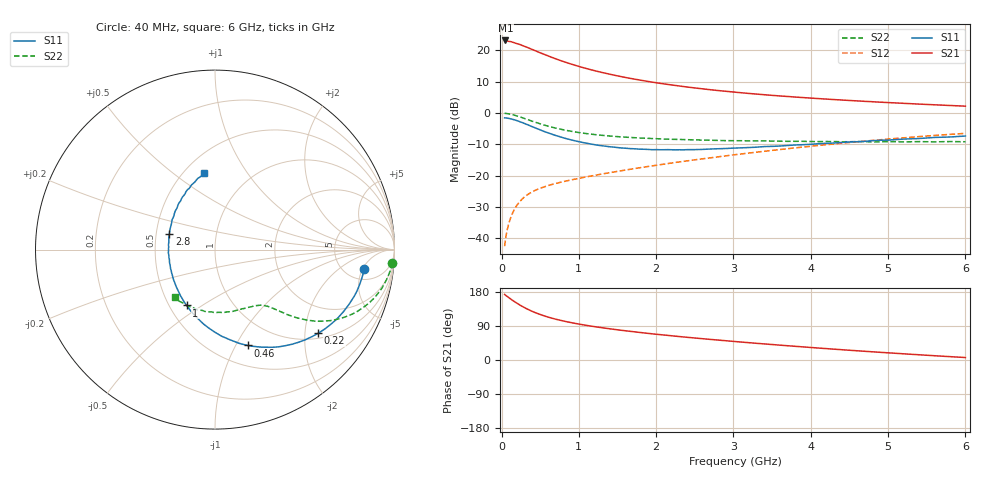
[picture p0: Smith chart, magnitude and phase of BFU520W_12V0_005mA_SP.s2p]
! Filename:  P:\Prog\Test\Noise\ATS_data\Testdata_Net\Run2\BFU520W_APM2013_06_A05_12p0V_005mA_SP_CM01_D.s2p
! Date/Time: Tue 26/Mar/2013 18:01:43
! BFU520W_APM2013_06_A05_12p0V_1to20mA_SP_CM01_Bias4_R.s2p
! MDIF S-parameter v. bias file
! BFU520W_APM2013_06_A05_12p0V_1to20mA_SP_CM01
! Date/time Thu Mar 21 16:35:01 2013
! VAR V_out= 12.0010
! VAR I_out= 5.0050
! VAR V_in= 0.8122
! VAR I_in= 0.0494
! Device data file deembeded for feedlines and parallel
! Original file: \Run2\BFU520W_APM2013_06_A05_12p0V_005mA_SP_CM01_R.s2p
! Feed-files: PR019V01_070313_Feed1.s2p, PR019V01_070313_Feed2.s2p
! Parallel-file: PR019V01_070313_Par.s2p
# MHz S MA R 50
!  Freq-MHz  S11-mag  S11-arg  S21-mag  S21-arg  S12-mag  S12-arg  S22-mag  S22-arg
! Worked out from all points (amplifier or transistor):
!   98 points, 40 MHz to 6 GHz, reference 50 ohm
!   highest |S21| = 23.2 dB at 50 MHz (marker M1)
!   |S21| within 3 dB of that: start of sweep to 409.2 MHz
!   unconditionally stable (mu >= 1): 1.889 GHz to 3.053 GHz
!   at 300 MHz: K = 0.32, MSG = 24.0 dB, |S12| = -26.8 dB
!   at 1.6 GHz: K = 0.97, MSG = 14.8 dB, |S12| = -18.2 dB
!   at 6 GHz: K = 0.86, MSG = 4.3 dB, |S12| = -6.5 dB
!   S11 on the Smith chart (normalised r, x): 40 MHz: 7.33, -5.42; 220 MHz: 1.13, -2.34; 460 MHz: 0.71, -1.12; 1 GHz: 0.61, -0.43; 2.8 GHz: 0.59, +0.11; 6 GHz: 0.63, +0.65
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40  0.8386 -7.5  14.41 173.1  0.007489 83.9  0.9894 -4.3
50  0.836 -9.3  14.42 171.4  0.009267 83.6  0.9873 -5.5
60  0.8331 -11.2  14.2 169.7  0.01116 82.6  0.984 -6.7
120  0.8065 -22.2  13.81 160.7  0.02159 77.6  0.9552 -12.9
160  0.7831 -29.1  13.32 155.2  0.02801 74.2  0.929 -16.7
220  0.7405 -39.0  12.64 147.2  0.03645 70.0  0.8814 -21.8
260  0.7105 -45.1  12.11 142.4  0.04146 67.4  0.8494 -24.8
320  0.663 -53.9  11.35 135.8  0.04807 64.3  0.8 -28.6
380  0.6183 -61.6  10.55 130.0  0.05365 61.8  0.7533 -31.7
460  0.5638 -71.2  9.606 123.2  0.06012 59.5  0.6986 -34.8
550  0.5081 -80.8  8.67 116.5  0.06613 57.8  0.6436 -37.5
700  0.4385 -94.5  7.353 107.7  0.07502 56.4  0.5753 -40.6
850  0.3868 -106.5  6.338 100.7  0.08299 56.1  0.5253 -42.5
1000  0.3489 -117.0  5.559 94.8  0.09064 56.5  0.4884 -43.9
1050  0.3391 -120.3  5.334 93.0  0.09317 56.7  0.4786 -44.4
1450  0.2859 -143.8  4.042 81.0  0.1144 58.4  0.4247 -47.7
2050  0.2594 -171.7  2.98 67.0  0.1496 60.2  0.3873 -53.6
2800  0.2691 161.4  2.288 52.6  0.1998 60.1  0.3655 -64.0
3100  0.2782 152.6  2.108 47.4  0.2222 59.4  0.3615 -68.5
4100  0.3237 129.6  1.702 31.5  0.3037 54.8  0.3499 -87.0
5200  0.3836 109.9  1.429 16.3  0.4021 46.7  0.346 -110.7
6000  0.4293 97.9  1.288 6.5  0.4739 39.3  0.3478 -130.4
